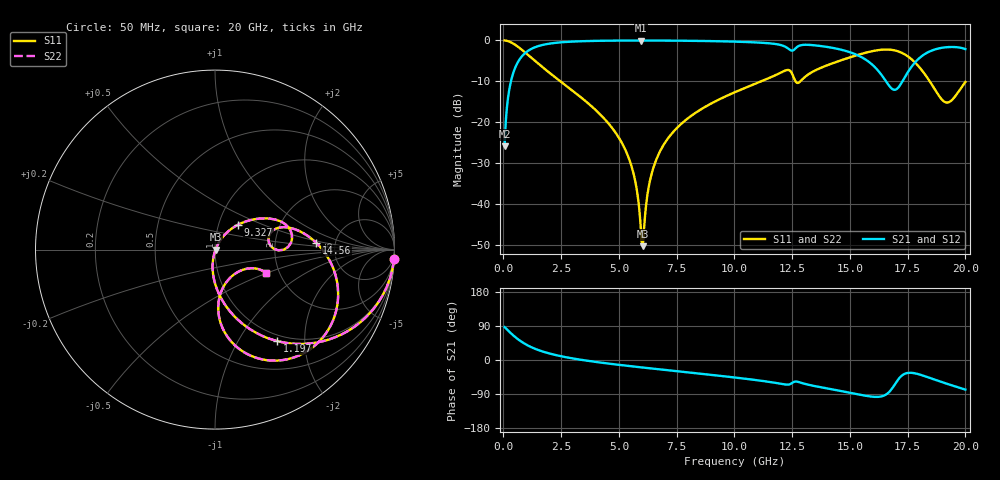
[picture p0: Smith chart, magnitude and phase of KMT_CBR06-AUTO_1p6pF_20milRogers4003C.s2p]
! Data measured by Modelithics Inc. support@modelithics.com 813-866-6335
! KEMET CBR06-AUTO 1.6pF, Pad Width= 0.851mm, Pad Length= 0.64mm, Pad Gap= 0.62mm, 20mil Rogers 4003C substrate Data, January 2022
# hz S ma R 50
! 2 Port Network Data from SP1.SP block
! freq  magS11  angS11  magS21  angS21  magS12  angS12  magS22  angS22
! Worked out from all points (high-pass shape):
!   401 points, 50 MHz to 20 GHz, reference 50 ohm
!   highest |S21| = -0.03 dB at 5.935 GHz (marker M1); lowest = -25.8 dB at 50 MHz (marker M2)
!   |S21| within 3 dB of the highest: 950.6 MHz to 15.08 GHz (14.12 GHz wide, 176 % of centre); 18.33 GHz to end of sweep
!   lowest |S11| = -50.2 dB at 6.035 GHz (marker M3), VSWR 1.01, Z = 50.3 - j0.00311 ohm
!   |S11| at or under -10 dB: 2.469 GHz to 11.15 GHz (8.684 GHz wide, 127 % of centre); 12.65 GHz to 12.85 GHz (201.6 MHz wide, 1.58 % of centre); 18.46 GHz to end of sweep
!   |S22| runs from -50.2 to 0.0 dB; largest |S21 - S12| = 0
!   S11 on the Smith chart (normalised r, x): 50 MHz: 1, -37; 1.197 GHz: 0.90, -1.49; 9.327 GHz: 1.24, +0.36; 14.56 GHz: 3.55, +0.39; 20 GHz: 1.70, -0.49
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5e7  0.9987 -3.1  0.05127 86.9  0.05127 86.9  0.9987 -3.1
2.495e8  0.9685 -15.2  0.2484 74.8  0.2484 74.8  0.9685 -15.2
4.49e8  0.907 -26.3  0.4202 63.6  0.4202 63.6  0.907 -26.3
1.197125e9  0.6166 -55.8  0.7857 34.1  0.7857 34.1  0.6166 -55.8
3.391625e9  0.1983 -89.1  0.9777 0.2  0.9777 0.2  0.1983 -89.1
5.237e9  0.04887 -101.3  0.9959 -14.5  0.9959 -14.5  0.04887 -101.3
5.685875e9  0.02038 -99.6  0.9968 -17.6  0.9968 -17.6  0.02038 -99.6
5.93525e9  0.005739 -79.1  0.9969 -19.2  0.9969 -19.2  0.005739 -79.1
6.035e9  0.003088 -0.6  0.9969 -19.9  0.9969 -19.9  0.003088 -0.6
6.33425e9  0.01891 59.0  0.9966 -21.9  0.9966 -21.9  0.01891 59.0
6.73325e9  0.04176 61.2  0.9958 -24.5  0.9958 -24.5  0.04176 61.2
9.32675e9  0.1898 47.1  0.9767 -41.4  0.9767 -41.4  0.1898 47.1
1.0025e10  0.2337 42.3  0.966 -46.2  0.966 -46.2  0.2337 42.3
1.256862e10  0.3522 -0.7  0.7645 -58.0  0.7645 -58.0  0.3522 -0.7
1.336662e10  0.4113 17.7  0.8766 -67.4  0.8766 -67.4  0.4113 17.7
1.456362e10  0.5653 3.8  0.7773 -81.3  0.7773 -81.3  0.5653 3.8
1.586038e10  0.7278 -19.5  0.5364 -96.1  0.5364 -96.1  0.7278 -19.5
1.670825e10  0.7724 -43.1  0.2777 -83.9  0.2777 -83.9  0.7724 -43.1
1.74065e10  0.6668 -66.6  0.367 -35.6  0.367 -35.6  0.6668 -66.6
1.825438e10  0.3838 -86.4  0.6851 -43.0  0.6851 -43.0  0.3838 -86.4
1.915212e10  0.1754 -57.3  0.8244 -61.8  0.8244 -61.8  0.1754 -57.3
2e10  0.3117 -24.6  0.7818 -78.1  0.7818 -78.1  0.3117 -24.6
